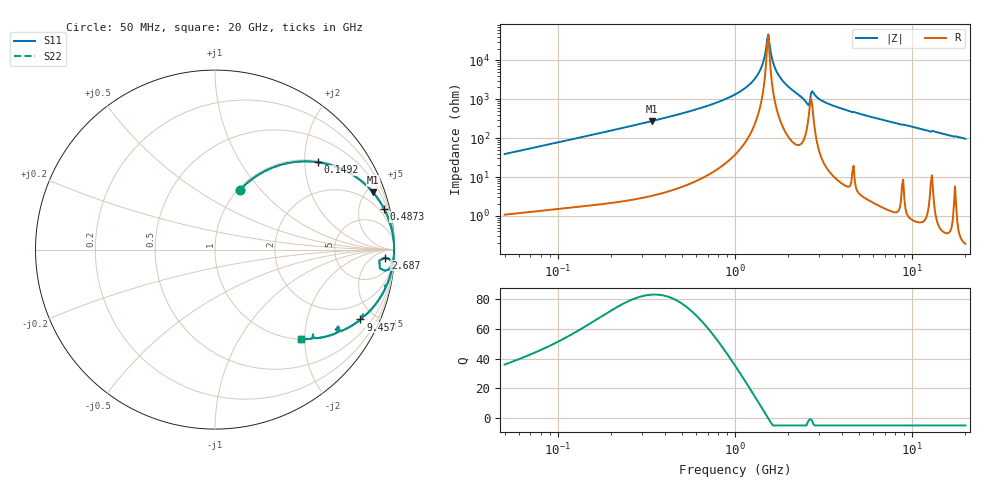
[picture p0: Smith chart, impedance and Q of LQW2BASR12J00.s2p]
!Murata Part Number: LQW2BASR12J00
!These Parameters are Measured in Series Mode Connection
!  o--[Z]--o
!Port1  Port2
!  o-------o
!Freq. Start=50[MHz] Stop=20[GHz], 401[Steps]
# Hz S RI R 50
!Freq.(Hz) S11(Real) S11(Imag) S21(Real) S21(Imag) S12(Real) S12(Imag) S22(Real) S22(Imag)
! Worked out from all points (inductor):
!   401 points, 50 MHz to 20 GHz, reference 50 ohm
!   read as one part in series: L = 124 nH near 51.52 MHz
!   highest Q = 83.2 at 340.1 MHz (marker M1), where L = 129 nH
!   self-resonance near 1.521 GHz
!   S11 on the Smith chart (normalised r, x): 50 MHz: 1.02, +0.78; 149.2 MHz: 1.04, +2.32; 487.3 MHz: 1.11, +8.31; 2.687 GHz: 21, -19; 9.457 GHz: 1.02, -4.15; 20 GHz: 1.00, -1.93
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5e7  0.1387 0.332  0.8613 -0.332  0.8613 -0.332  0.1387 0.332
1.364002e8  0.5289 0.491  0.4711 -0.491  0.4711 -0.491  0.5289 0.491
1.492265e8  0.5732 0.4868  0.4268 -0.4868  0.4268 -0.4868  0.5732 0.4868
3.401177e8  0.8801 0.3189  0.1199 -0.3189  0.1199 -0.3189  0.8801 0.3189
3.721004e8  0.8992 0.2951  0.1008 -0.2951  0.1008 -0.2951  0.8992 0.2951
4.872511e8  0.9427 0.2262  0.0573 -0.2262  0.0573 -0.2262  0.9427 0.2262
1e9  0.9922 0.0749  0.00779 -0.0749  0.00779 -0.0749  0.9922 0.0749
1.179116e9  0.9958 0.0457  0.00416 -0.0457  0.00416 -0.0457  0.9958 0.0457
1.329223e9  0.9973 0.025  0.00267 -0.025  0.00267 -0.025  0.9973 0.025
1.411297e9  0.9977 0.0147  0.00226 -0.0147  0.00226 -0.0147  0.9977 0.0147
1.498439e9  0.9979 0.00447  0.00207 -0.00447  0.00207 -0.00447  0.9979 0.00447
1.544007e9  0.9979 -0.000688  0.00206 0.000688  0.00206 0.000688  0.9979 -0.000688
1.567309e9  0.9979 -0.00327  0.00208 0.00327  0.00208 0.00327  0.9979 -0.00327
1.689197e9  0.9976 -0.0163  0.00237 0.0163  0.00237 0.0163  0.9976 -0.0163
1.848039e9  0.9967 -0.0324  0.00327 0.0324  0.00327 0.0324  0.9967 -0.0324
2.531158e9  0.9645 -0.1132  0.0355 0.1132  0.0355 0.1132  0.9645 -0.1132
2.687447e9  0.9486 -0.0443  0.0514 0.0443  0.0514 0.0443  0.9486 -0.0443
2.728004e9  0.97 -0.0526  0.03 0.0526  0.03 0.0526  0.97 -0.0526
3.736399e9  0.9739 -0.1527  0.0261 0.1527  0.0261 0.1527  0.9739 -0.1527
7.442007e9  0.8758 -0.3272  0.1242 0.3272  0.1242 0.3272  0.8758 -0.3272
9.457416e9  0.8106 -0.3894  0.1894 0.3894  0.1894 0.3894  0.8106 -0.3894
2e10  0.4811 -0.4987  0.5189 0.4987  0.5189 0.4987  0.4811 -0.4987
